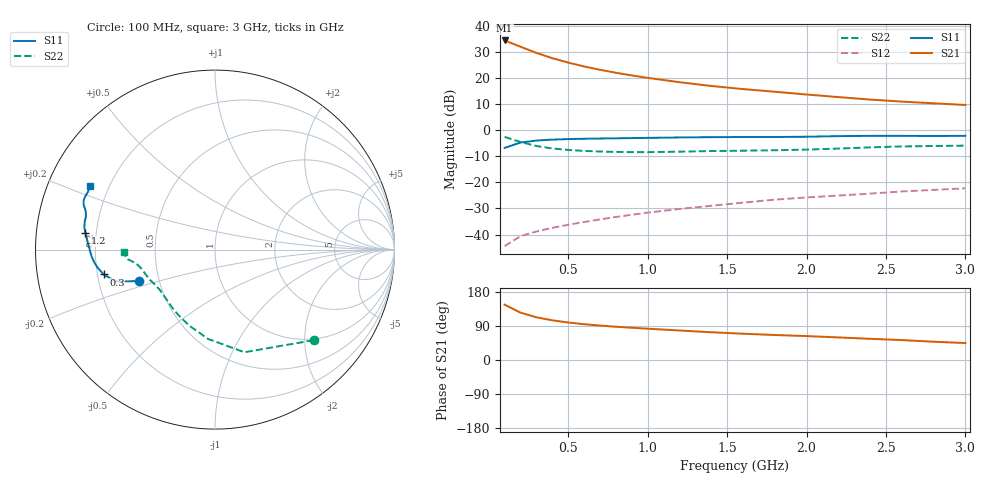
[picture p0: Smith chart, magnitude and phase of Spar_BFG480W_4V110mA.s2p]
! Filename: 4110BFG480.001
! Title: BFG480W
! Bias: Vce=4V; Ic=110mA
! Company: NXP Semiconductors NL
! User: Quality&Reliability T&D
! Measure time: 10 Nov 1999 / 12:04:13
#  MHz  S  MA  R 50
! Freq  S11  S21  S12  S22  :
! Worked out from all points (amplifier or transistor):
!   20 points, 100 MHz to 3 GHz, reference 50 ohm
!   highest |S21| = 34.5 dB at 100 MHz (marker M1)
!   |S21| within 3 dB of that: start of sweep to 225.2 MHz
!   unconditionally stable (mu >= 1): 679.1 MHz to end of sweep
!   at 400 MHz: K = 0.84, MSG = 32.5 dB, |S12| = -37.4 dB
!   at 1.2 GHz: K = 1.08, MAG = 22.6 dB, |S12| = -30.2 dB
!   at 3 GHz: K = 1.05, MAG = 14.6 dB, |S12| = -22.2 dB
!   S11 on the Smith chart (normalised r, x): 100 MHz: 0.38, -0.17; 300 MHz: 0.23, -0.10; 1.2 GHz: 0.16, +0.06; 3 GHz: 0.13, +0.24
100  0.4591 -157.5  52.82 146.1  0.00599 68.9  0.7461 -42.6
200  0.5815 -162.2  40.04 125.0  0.009324 60.6  0.5951 -74.0
300  0.6352 -167.4  30.5 112.8  0.01143 60.1  0.4994 -94.4
400  0.6621 -171.3  24.16 104.8  0.01347 62.3  0.448 -108.4
500  0.6778 -174.3  19.87 99.0  0.01542 64.4  0.4196 -118.5
600  0.688 -176.7  16.76 94.5  0.0174 66.3  0.4026 -126.0
700  0.695 -178.9  14.48 90.9  0.01953 68.3  0.3914 -131.8
800  0.7011 179.1  12.7 87.8  0.02175 70.1  0.3845 -136.6
900  0.7088 177.3  11.28 85.1  0.02391 71.8  0.3812 -140.8
1000  0.7149 175.6  10.14 82.6  0.02634 72.7  0.3811 -144.5
1200  0.7284 172.6  8.363 77.9  0.03095 74.2  0.3886 -150.5
1400  0.7379 170.4  7.078 73.2  0.03564 75.0  0.3995 -155.0
1600  0.7426 168.1  6.172 69.4  0.04098 75.7  0.4061 -158.4
1800  0.7423 165.5  5.486 66.0  0.0467 76.2  0.414 -162.0
2000  0.7524 163.3  4.855 63.1  0.05151 76.7  0.4262 -166.3
2200  0.7724 161.2  4.333 59.6  0.05597 76.6  0.4457 -170.0
2400  0.7818 159.5  3.883 55.9  0.06094 76.0  0.4703 -172.3
2600  0.7813 157.8  3.549 52.6  0.06712 75.3  0.49 -173.7
2800  0.7774 155.6  3.29 48.2  0.07183 73.9  0.4995 -175.5
3000  0.7822 152.9  3.055 44.8  0.07722 73.1  0.5076 -178.3
